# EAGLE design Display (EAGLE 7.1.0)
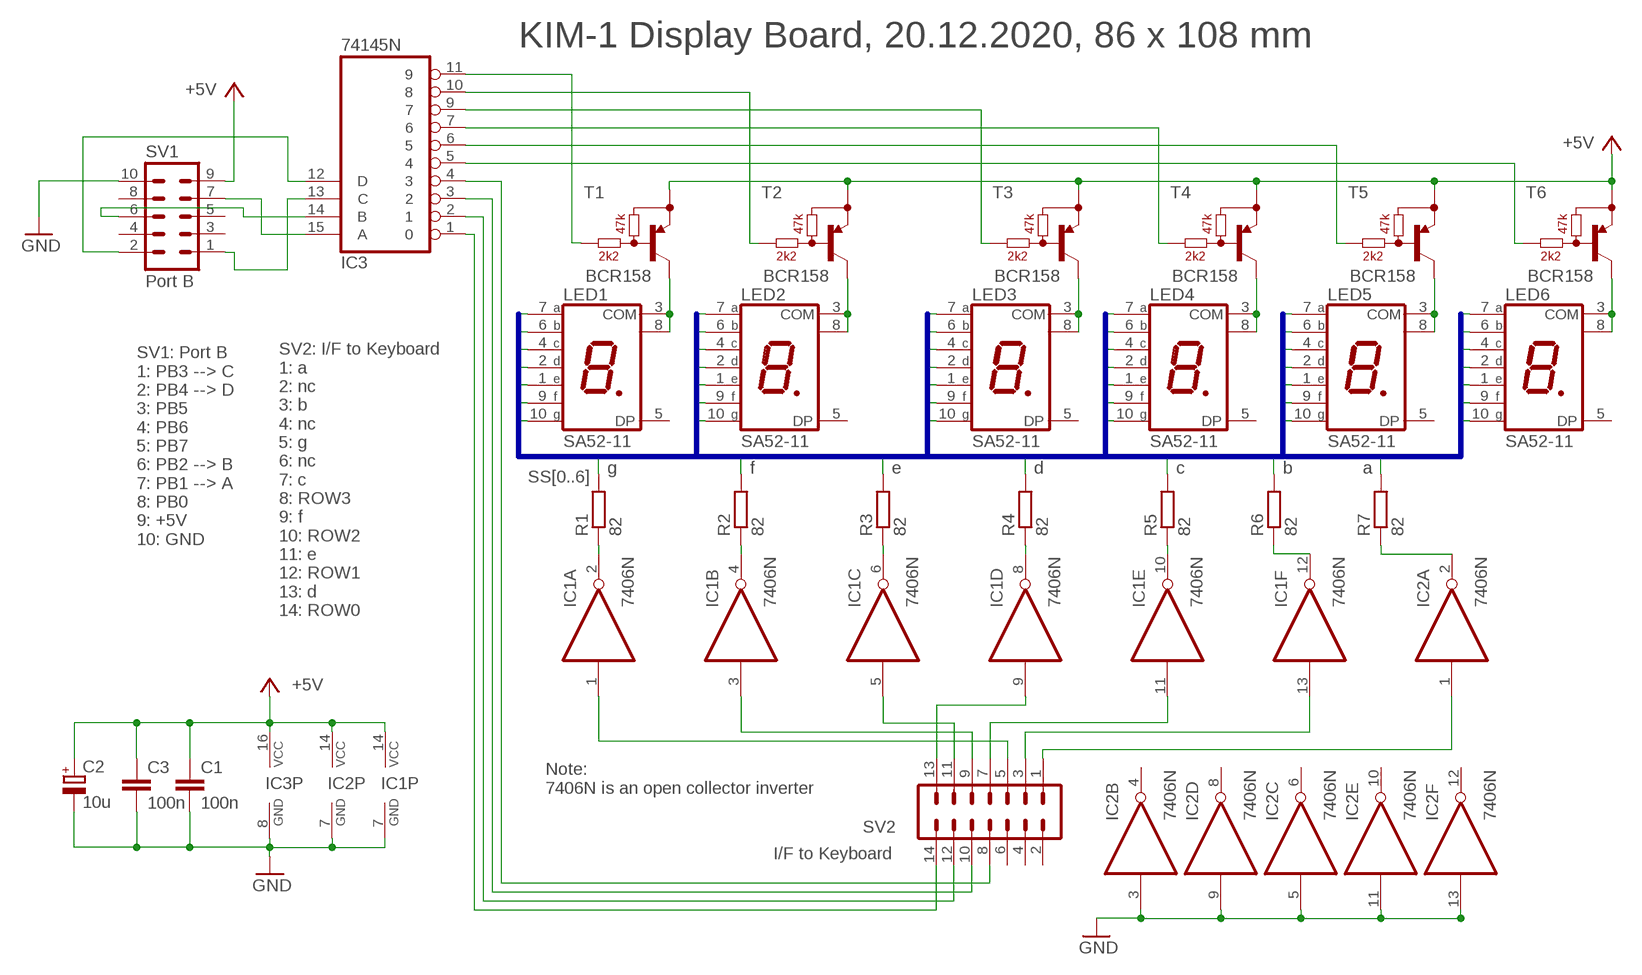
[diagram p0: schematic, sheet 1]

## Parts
C1  100n  C-EUC1206  [C1206]
C2  10u  CPOL-EUE2.5-6  [E2,5-6]
C3  100n  C-EUC1206  [C1206]
IC1  7406N  [DIL14]
IC2  7406N  [DIL14]
IC3  74145N  [DIL16]
LED1  SA52-11  7-SEG_SA52-11  [SA52-11]
LED2  SA52-11  7-SEG_SA52-11  [SA52-11]
LED3  SA52-11  7-SEG_SA52-11  [SA52-11]
LED4  SA52-11  7-SEG_SA52-11  [SA52-11]
LED5  SA52-11  7-SEG_SA52-11  [SA52-11]
LED6  SA52-11  7-SEG_SA52-11  [SA52-11]
R1  82  R-EU_R1206  [R1206]
R2  82  R-EU_R1206  [R1206]
R3  82  R-EU_R1206  [R1206]
R4  82  R-EU_R1206  [R1206]
R5  82  R-EU_R1206  [R1206]
R6  82  R-EU_R1206  [R1206]
R7  82  R-EU_R1206  [R1206]
SV1  Port B  ML10  [ML10]
SV2  I/F to Keyboard  ML14  [ML14]
T1  BCR158  BCR158-W  [SOT23-W_INFINEON]
T2  BCR158  BCR158-W  [SOT23-W_INFINEON]
T3  BCR158  BCR158-W  [SOT23-W_INFINEON]
T4  BCR158  BCR158-W  [SOT23-W_INFINEON]
T5  BCR158  BCR158-W  [SOT23-W_INFINEON]
T6  BCR158  BCR158-W  [SOT23-W_INFINEON]

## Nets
+5V: C1.1 C2.+ C3.1 IC1.14(P:VCC) IC2.14(P:VCC) IC3.16(VCC) SV1.9 T1.2(E) T2.2(E) T3.2(E) T4.2(E) T5.2(E) T6.2(E)
GND: C1.2 C2.- C3.2 IC1.7(P:GND) IC2.3(B:I) IC2.5(C:I) IC2.7(P:GND) IC2.9(D:I) IC2.11(E:I) IC2.13(F:I) IC3.8(GND) SV1.10
N$1: LED6.3(COM) LED6.8(COM) T6.3(C)
N$2: LED5.3(COM) LED5.8(COM) T5.3(C)
N$3: LED3.3(COM) LED3.8(COM) T3.3(C)
N$4: LED2.3(COM) LED2.8(COM) T2.3(C)
N$5: LED1.3(COM) LED1.8(COM) T1.3(C)
N$6: LED4.3(COM) LED4.8(COM) T4.3(C)
N$7: IC1.2(A:O) R1.1
N$8: IC1.4(B:O) R2.1
N$9: IC1.6(C:O) R3.1
N$10: IC1.8(D:O) R4.1
N$11: IC1.10(E:O) R5.1
N$12: IC1.12(F:O) R6.1
N$13: IC2.2(A:O) R7.1
N$14: IC3.11 T1.1(B)
N$15: IC3.10 T2.1(B)
N$16: IC3.9 T3.1(B)
N$17: IC3.7 T4.1(B)
N$18: IC3.6 T5.1(B)
N$19: IC3.5 T6.1(B)
N$20: IC1.1(A:I) SV2.5
N$21: IC1.3(B:I) SV2.9
N$22: IC1.5(C:I) SV2.11
N$23: IC1.9(D:I) SV2.13
N$24: IC1.11(E:I) SV2.7
N$25: IC1.13(F:I) SV2.3
N$26: IC2.1(A:I) SV2.1
N$27: IC3.1 SV2.14
N$28: IC3.2 SV2.12
N$29: IC3.3 SV2.10
N$30: IC3.4 SV2.8
N$31: IC3.15(A) SV1.7
N$36: IC3.14(B) SV1.6
N$37: IC3.13(C) SV1.1
N$38: IC3.12(D) SV1.2
SS0: LED1.7(A) LED2.7(A) LED3.7(A) LED4.7(A) LED5.7(A) LED6.7(A) R7.2
SS1: LED1.6(B) LED2.6(B) LED3.6(B) LED4.6(B) LED5.6(B) LED6.6(B) R6.2
SS2: LED1.4(C) LED2.4(C) LED3.4(C) LED4.4(C) LED5.4(C) LED6.4(C) R5.2
SS3: LED1.2(D) LED2.2(D) LED3.2(D) LED4.2(D) LED5.2(D) LED6.2(D) R4.2
SS4: LED1.1(E) LED2.1(E) LED3.1(E) LED4.1(E) LED5.1(E) LED6.1(E) R3.2
SS5: LED1.9(F) LED2.9(F) LED3.9(F) LED4.9(F) LED5.9(F) LED6.9(F) R2.2
SS6: LED1.10(G) LED2.10(G) LED3.10(G) LED4.10(G) LED5.10(G) LED6.10(G) R1.2
Unconnected: IC2.4(B:O) IC2.6(C:O) IC2.8(D:O) IC2.10(E:O) IC2.12(F:O) LED1.5(DP) LED2.5(DP) LED3.5(DP) LED4.5(DP) LED5.5(DP) LED6.5(DP) SV1.3 SV1.4 SV1.5 SV1.8 SV2.2 SV2.4 SV2.6

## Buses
SS[0..6]

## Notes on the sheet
- KIM-1 Display Board, 20.12.2020, 86 x 108 mm
- g | f | e | d | c | b | a
- SV1: Port B
  1: PB3 --> C
  2: PB4 --> D
  3: PB5
  4: PB6
  5: PB7
  6: PB2 --> B
  7: PB1 --> A
  8: PB0
  9: +5V
  10: GND
- SV2: I/F to Keyboard
  1: a
  2: nc
  3: b
  4: nc
  5: g
  6: nc
  7: c
  8: ROW3
  9: f
  10: ROW2
  11: e
  12: ROW1
  13: d
  14: ROW0
- Note:
  7406N is an open collector inverter

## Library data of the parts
C1 C3 = rcl:C-EU: CAPACITOR, European symbol
C2 = rcl:CPOL-EU: POLARIZED CAPACITOR, European symbol
IC1 IC2 = 74xx-eu:74*06: Hex INVERTER, open collector high-voltage output
IC3 = 74xx-eu:74*145: BCD to decimal DECODER/DRIVER
LED1-LED6 = display-kingbright:7-SEG_: Kingbright 14.2mm (0.56 INCH) SINGLE DIGIT NUMERIC DUISPLAY Source: SA56-11EWA(Ver1189471036.pdf; OC_FARNELL: unknown; OC_NEWARK: unknown
R1-R7 = rcl:R-EU_: RESISTOR, European symbol
SV1 = con-harting-ml:ML10: HARTING; OC_FARNELL: unknown; OC_NEWARK: unknown
SV2 = con-harting-ml:ML14: HARTING; OC_FARNELL: unknown; OC_NEWARK: unknown
T1-T6 = digital-transistors-1:BCR158: PNP Silicon Digital Transistor 50V 0,1A 0,2W

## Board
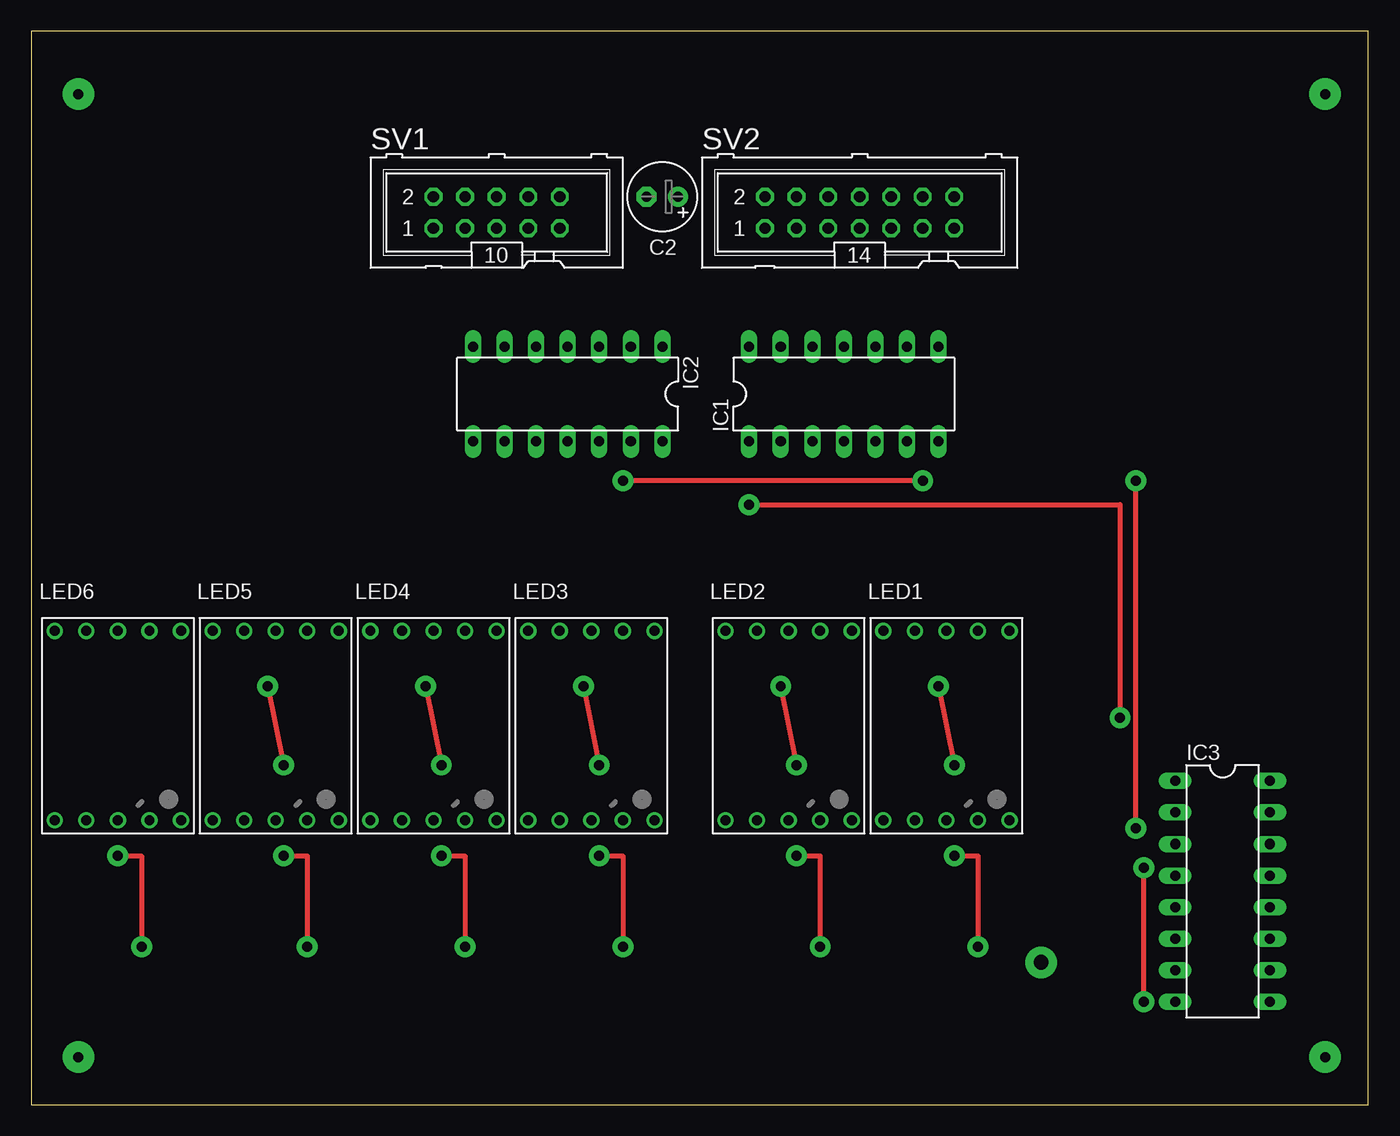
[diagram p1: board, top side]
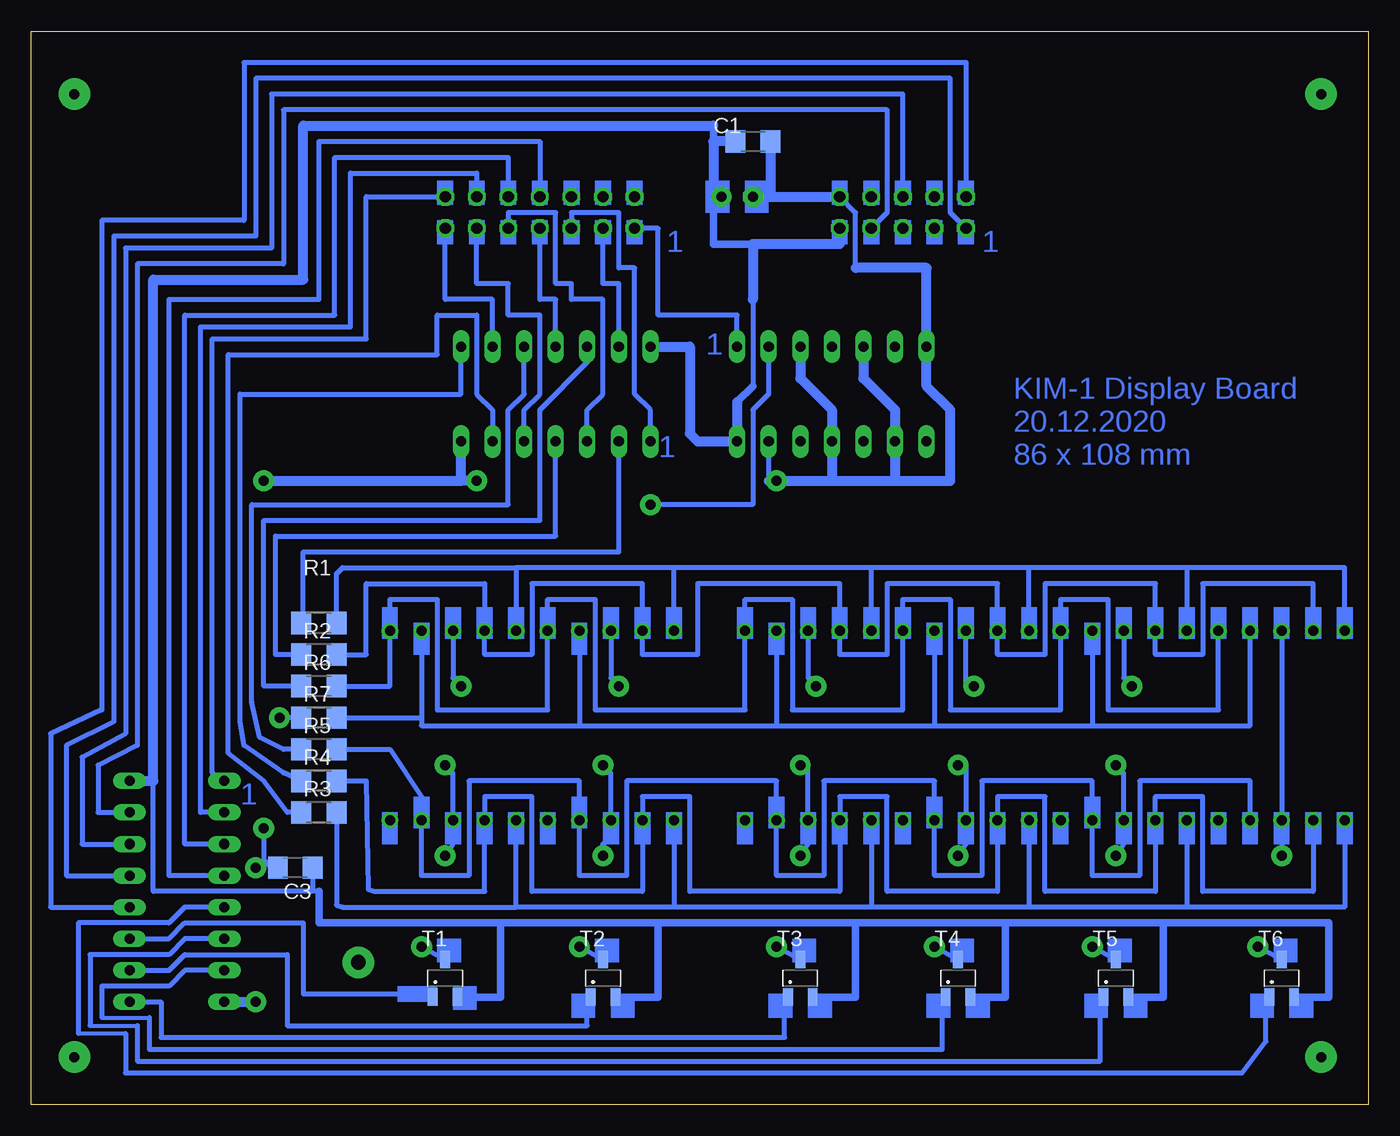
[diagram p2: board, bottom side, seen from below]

Size 107.62 x 86.35 mm. Coordinates in mm from the lower left corner, seen from the top.
Outline: 0,0 107.62,0 107.62,86.35 0,86.35 0,0
Copper layers (1*16): Top 0.035mm / dielectric 1.5mm / Bottom 0.035mm
Design rules "default": minimum track width 10mil, minimum drill 24mil, track to track 8mil, track to pad 8mil, pad to pad 8mil, via to via 8mil, smd to smd 8mil, copper to edge 40mil, drill to drill 8mil, minimum pad ring 10mil, minimum via ring 8mil, stop-mask expansion 4mil, vias tented up to drill 0mil, thermal gap 10mil

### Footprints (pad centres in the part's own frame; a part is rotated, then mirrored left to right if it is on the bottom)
C1206 = smd 1.6 x 1.8: 1 -1.4,0; 2 1.4,0
E2,5-6 = drill 0.813 pad 1.6: + -1.27,0 | drill 0.813 pad 1.6 octagon: - 1.27,0
DIL14 = drill 0.813 long: 1 -7.62,-3.81; 2 -5.08,-3.81; 3 -2.54,-3.81; 4 0,-3.81; 5 2.54,-3.81; 6 5.08,-3.81; 7 7.62,-3.81; 8 7.62,3.81; 9 5.08,3.81; 10 2.54,3.81; 11 0,3.81; 12 -2.54,3.81; 13 -5.08,3.81; 14 -7.62,3.81
DIL16 = drill 0.813 long: 1 -8.89,-3.81; 2 -6.35,-3.81; 3 -3.81,-3.81; 4 -1.27,-3.81; 5 1.27,-3.81; 6 3.81,-3.81; 7 6.35,-3.81; 8 8.89,-3.81; 9 8.89,3.81; 10 6.35,3.81; 11 3.81,3.81; 12 1.27,3.81; 13 -1.27,3.81; 14 -3.81,3.81; 15 -6.35,3.81; 16 -8.89,3.81
SA52-11 = drill 0.8: 1 -5.08,-7.62; 2 -2.54,-7.62; 3 0,-7.62; 4 2.54,-7.62; 5 5.08,-7.62; 6 5.08,7.62; 7 2.54,7.62; 8 0,7.62; 9 -2.54,7.62; 10 -5.08,7.62
R1206 = smd 1.6 x 1.803: 1 -1.422,0; 2 1.422,0
ML10 = drill 0.914 octagon: 1 -5.08,-1.27; 2 -5.08,1.27; 3 -2.54,-1.27; 4 -2.54,1.27; 5 0,-1.27; 6 0,1.27; 7 2.54,-1.27; 8 2.54,1.27; 9 5.08,-1.27; 10 5.08,1.27
ML14 = drill 0.914 octagon: 1 -7.62,-1.27; 2 -7.62,1.27; 3 -5.08,-1.27; 4 -5.08,1.27; 5 -2.54,-1.27; 6 -2.54,1.27; 7 0,-1.27; 8 0,1.27; 9 2.54,-1.27; 10 2.54,1.27; 11 5.08,-1.27; 12 5.08,1.27; 13 7.62,-1.27; 14 7.62,1.27
SOT23-W_INFINEON = smd 0.8 x 1.4: 1 -1,-1.5; 2 1,-1.5; 3 0,1.5

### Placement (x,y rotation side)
C1  49.53,77.47 0 bottom
C2  50.8,73.03 180 top
C3  86.36,19.05 180 bottom
IC1  65.41,57.15 0 top
IC2  43.18,57.15 180 top
IC3  95.89,17.14 270 top
LED1  73.66,30.48 0 top
LED2  60.96,30.48 0 top
LED3  45.09,30.48 0 top
LED4  32.38,30.48 0 top
LED5  19.68,30.48 0 top
LED6  6.99,30.48 0 top
R1  84.45,38.73 0 bottom
R2  84.45,36.2 0 bottom
R3  84.45,23.5 0 bottom
R4  84.45,26.04 0 bottom
R5  84.45,28.57 0 bottom
R6  84.45,33.66 0 bottom
R7  84.45,31.11 0 bottom
SV1  37.47,71.75 0 top
SV2  66.67,71.75 0 top
T1  74.3,10.16 0 bottom
T2  61.59,10.16 0 bottom
T3  45.72,10.16 0 bottom
T4  33.02,10.16 0 bottom
T5  20.32,10.16 0 bottom
T6  6.99,10.16 0 bottom

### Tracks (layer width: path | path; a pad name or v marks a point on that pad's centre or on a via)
+5V
  Bottom 0.406: T6.2 5.99,8.62 | T1.2 73.3,8.62 | T2.2 60.59,8.62 | T5.2 18.68,8.62 | T4.2 31.39,8.62 | T3.2 44.72,8.62 | 51.44,53.34 IC2.14 | 49.53,64.77 49.53,57.78 | 84.45,17.14 85.09,17.14 | 85.09,17.14 97.79,17.14 97.79,26.04 | C3.1 84.96,17.27 85.09,17.14
  Bottom 0.61: 5.99,8.62 3.17,8.62 3.17,14.61 16.51,14.61 | 16.51,14.61 29.21,14.61 | 29.21,14.61 41.27,14.61 | 41.27,14.61 57.15,14.61 | 57.15,14.61 69.85,14.61 | 73.3,8.62 69.85,8.62 69.85,14.61 | 60.59,8.62 57.15,8.62 57.15,14.61 | 18.68,8.62 16.51,8.62 16.51,14.61 | 31.39,8.62 29.21,8.62 29.21,14.61 | 44.72,8.62 41.27,8.62 41.27,14.61 | 69.85,14.61 84.45,14.61 84.45,17.14 | 52.7,78.74 52.7,77.47 | 49.53,69.22 52.7,69.22 52.7,73.03 C2.+ | 49.53,57.78 50.8,56.52 | 50.8,53.98 51.44,53.34
  Bottom 0.813: IC3.16 97.79,26.04 97.79,66.36 85.72,66.36 85.72,78.74 52.7,78.74 | 52.7,73.03 52.7,77.47 C1.1 | 49.53,64.77 49.53,69.22 42.55,69.22 SV1.9 | IC1.14 54.61,60.96 54.61,53.98 53.98,53.34 51.44,53.34 | 50.8,56.52 50.8,53.98
GND  (via drill 0.8 pad 1.68)
  Top 0.406: v71.75,50.16 v47.62,50.16 | v89.53,8.26 v89.53,19.05 | v88.9,22.23 v88.9,50.16
  Bottom 0.406: IC2.13 48.26,50.16 | 41.27,67.31 41.27,71.75 SV1.10 | v88.9,22.23 88.9,19.68 | 88.9,19.68 v89.53,19.05 | C3.2 88.27,19.05 88.9,19.68
  Bottom 0.61: C2.- 48.26,73.03 48.13,73.16
  Bottom 0.813: v88.9,50.16 73.03,50.16 | 73.03,50.16 IC1.7 | IC3.8 v89.53,8.26 | v71.75,50.16 73.03,50.16 | 43.18,50.16 v47.62,50.16 48.26,50.16 | 43.18,50.16 38.1,50.16 | 38.1,50.16 33.66,50.16 33.66,55.88 35.56,57.78 IC2.7 35.56,67.31 41.27,67.31 | 48.26,73.03 SV1.10 | C1.2 48.13,73.16 | 43.18,50.16 IC2.11 43.18,55.88 45.72,58.42 IC2.3 | 38.1,50.16 IC2.9 38.1,55.88 40.64,58.42 IC2.5
N$1  (via drill 0.8 pad 1.68)
  Top 0.406: v6.99,20 8.89,20 v8.89,12.7
  Bottom 0.406: LED6.8 LED6.3 v6.99,20 | T6.3 v8.89,12.7
N$2  (via drill 0.8 pad 1.68)
  Top 0.406: v19.05,33.66 v20.32,27.3 | v20.32,20 22.23,20 v22.23,12.7
  Bottom 0.406: LED5.8 19.68,34.29 19.05,34.29 v19.05,33.66 | v20.32,27.3 20.32,26.67 19.68,26.67 LED5.3 19.68,20.95 v20.32,20 | T5.3 v22.23,12.7
N$3  (via drill 0.8 pad 1.68)
  Top 0.406: v44.45,33.66 v45.72,27.3 | v45.72,20 47.62,20 v47.62,12.7
  Bottom 0.406: LED3.8 45.09,34.29 44.45,34.29 v44.45,33.66 | v45.72,27.3 45.09,27.3 LED3.3 45.09,20.95 v45.72,20 | T3.3 v47.62,12.7
N$4  (via drill 0.8 pad 1.68)
  Top 0.406: v60.33,33.66 v61.59,27.3 | v61.59,20 63.5,20 v63.5,12.7
  Bottom 0.406: v61.59,27.3 61.59,26.67 60.96,26.67 LED2.3 60.96,21.59 61.59,20.95 v61.59,20 | LED2.8 60.96,34.29 60.33,34.29 v60.33,33.66 | T2.3 v63.5,12.7
N$5  (via drill 0.8 pad 1.68)
  Top 0.406: v73.03,33.66 v74.3,27.3 | v74.3,20 76.2,20 v76.2,12.7
  Bottom 0.406: LED1.8 73.66,34.29 73.03,34.29 v73.03,33.66 | v74.3,27.3 74.3,26.67 73.66,26.67 LED1.3 73.66,20.95 v74.3,20 | T1.3 v76.2,12.7
N$6  (via drill 0.8 pad 1.68)
  Top 0.406: v31.75,33.66 v33.02,27.3 | v33.02,20 34.92,20 v34.92,12.7
  Bottom 0.406: v31.75,33.66 32.38,33.66 LED4.8 | v33.02,27.3 32.38,27.3 LED4.3 32.38,20.95 v33.02,20 | T4.3 v34.92,12.7
N$7
  Bottom 0.406: R1.1 85.72,38.73 85.72,44.45 60.33,44.45 IC1.2
N$8
  Bottom 0.406: R2.1 87.95,36.2 87.95,45.72 65.41,45.72 IC1.4
N$9
  Bottom 0.406: R3.1 87,23.5 88.9,26.04 91.76,28.26 91.76,60.33 74.93,60.33 74.93,63.5 71.75,63.5 71.75,57.15 70.48,55.88 IC1.6
N$10
  Bottom 0.406: R4.1 87.31,26.67 90.49,28.89 90.81,30.8 90.81,57.15 73.03,57.15 IC1.8
N$11
  Bottom 0.406: R5.1 87.31,28.57 89.22,29.53 89.85,32.38 89.85,48.26 69.22,48.26 69.22,55.88 67.94,57.15 IC1.10
N$12
  Bottom 0.406: R6.1 88.9,33.66 88.9,46.99 66.67,46.99 66.67,55.88 62.87,59.69 IC1.12
N$13  (via drill 0.8 pad 1.68)
  Top 0.406: v57.78,48.26 87.63,48.26 v87.63,31.11
  Bottom 0.406: R7.1 v87.63,31.11 | IC2.2 48.26,57.15 49.53,55.88 49.53,48.26 v57.78,48.26
N$14
  Bottom 0.406: IC3.11 96.52,13.34 95.25,14.61 85.72,14.61 85.72,8.89 75.53,8.89 T1.1
N$15
  Bottom 0.406: IC3.10 96.52,10.79 95.25,12.06 87,12.06 87,6.35 62.87,6.35 62.87,8.39 T2.1
N$16
  Bottom 0.406: IC3.9 97.16,8.26 97.16,5.4 46.99,5.4 46.99,8.39 T3.1
N$17
  Bottom 0.305: 101.92,6.99 98.11,6.99
  Bottom 0.406: IC3.7 95.25,10.79 96.52,9.53 101.92,9.53 101.92,6.99 | 98.11,6.99 98.11,4.45 34.29,4.45 34.29,8.39 T4.1
N$18
  Bottom 0.305: 102.87,6.35 99.06,6.35
  Bottom 0.406: IC3.6 95.25,13.34 96.52,12.06 102.87,12.06 102.87,6.35 | 99.06,6.35 99.06,3.49 21.59,3.49 21.59,8.39 T5.1
N$19
  Bottom 0.305: 103.82,5.71 100.01,5.71
  Bottom 0.406: IC3.5 95.25,15.88 96.52,14.61 103.82,14.61 103.82,5.71 | 100.01,5.71 100.01,2.54 10.16,2.54 8.26,5.08 8.26,8.39 T6.1
N$20
  Bottom 0.406: IC1.1 57.78,55.88 59.05,57.15 59.05,67.31 60.33,67.31 60.33,71.75 64.14,71.75 SV2.5
N$21
  Bottom 0.406: IC1.3 62.87,55.88 61.59,57.15 61.59,64.77 64.14,64.77 64.14,66.04 65.41,66.04 65.41,71.75 69.22,71.75 SV2.9
N$22
  Bottom 0.406: IC1.5 67.94,55.88 66.67,57.15 66.67,63.5 69.22,63.5 69.22,66.04 71.75,66.04 SV2.11
N$23
  Bottom 0.406: IC1.9 70.48,64.77 74.3,64.77 SV2.13
N$24
  Bottom 0.406: IC1.11 65.41,64.77 66.67,64.77 SV2.7
N$25
  Bottom 0.406: IC1.13 60.33,66.04 61.59,66.04 SV2.3
N$26
  Bottom 0.406: IC2.1 50.8,63.5 57.15,63.5 57.15,70.48 SV2.1
N$27
  Bottom 0.406: IC3.1 93.03,26.67 93.03,61.59 80.64,61.59 80.64,73.03 SV2.14
N$28
  Bottom 0.406: IC3.2 93.98,23.5 93.98,62.55 81.92,62.55 81.92,74.93 71.75,74.93 SV2.12
N$29
  Bottom 0.406: IC3.3 95.25,20.95 95.25,63.5 83.19,63.5 83.19,76.2 69.22,76.2 SV2.10
N$30
  Bottom 0.406: IC3.4 96.52,18.41 96.52,64.77 84.45,64.77 84.45,77.47 66.67,77.47 SV2.8
N$31
  Bottom 0.406: IC3.15 102.23,23.5 102.23,27.3 99.06,28.89 99.06,67.63 87.31,67.63 87.31,80.01 38.73,80.01 38.73,71.75 SV1.7
N$32  (via drill 0.8 pad 2.54)
  other vias: 3.81,81.28
N$33  (via drill 0.8 pad 2.54)
  other vias: 104.14,81.28
N$34  (via drill 0.8 pad 2.54)
  other vias: 104.14,3.81
N$35  (via drill 0.8 pad 2.54)
  other vias: 3.81,3.81
N$36
  Bottom 0.406: IC3.14 103.5,20.95 103.5,27.94 100.01,29.84 100.01,68.9 88.27,68.9 88.27,81.28 37.47,81.28 SV1.6
N$37
  Bottom 0.406: IC3.13 104.78,18.41 104.78,28.89 100.97,30.8 100.97,69.85 89.53,69.85 89.53,82.55 33.66,82.55 33.66,71.75 SV1.1
N$38
  Bottom 0.406: IC3.12 106.05,15.88 106.05,29.84 101.92,31.75 101.92,71.12 90.49,71.12 90.49,83.82 32.38,83.82 SV1.2
N$39  (via drill 1.2 pad 2.54)
  other vias: 81.28,11.43
SS0
  Bottom 0.406: LED1.7 76.2,31.11 | 76.2,31.11 76.2,30.48 63.5,30.48 | 63.5,30.48 47.62,30.48 | 47.62,30.48 34.92,30.48 | 34.92,30.48 22.23,30.48 | 22.23,30.48 9.53,30.48 LED6.7 | LED5.7 22.23,30.48 | LED4.7 34.92,30.48 | LED3.7 47.62,30.48 | LED2.7 63.5,30.48 | R7.2 76.2,31.11
SS1
  Bottom 0.406: LED6.6 12.06,31.75 20.95,31.75 20.95,40.64 24.77,40.64 LED5.6 24.77,31.75 33.66,31.75 33.66,40.64 37.47,40.64 LED4.6 37.47,31.75 46.35,31.75 46.35,40.64 50.16,40.64 LED3.6 50.16,31.75 62.23,31.75 62.23,40.64 66.04,40.64 LED2.6 66.04,31.75 74.93,31.75 74.93,40.64 78.74,40.64 LED1.6 78.74,33.66 R6.2
SS2
  Bottom 0.406: LED6.4 9.53,26.04 18.41,26.04 18.41,18.41 22.23,18.41 LED5.4 22.23,26.04 31.11,26.04 31.11,18.41 34.92,18.41 LED4.4 34.92,26.04 43.81,26.04 43.81,18.41 47.62,18.41 LED3.4 47.62,26.04 59.69,26.04 59.69,18.41 63.5,18.41 LED2.4 63.5,26.04 72.39,26.04 72.39,18.41 76.2,18.41 LED1.4 76.2,24.77 78.74,28.57 R5.2
SS3
  Bottom 0.406: LED6.2 4.45,17.14 13.34,17.14 13.34,24.77 17.14,24.77 LED5.2 17.14,17.14 26.04,17.14 26.04,24.77 29.84,24.77 LED4.2 29.84,17.14 38.73,17.14 38.73,24.77 42.55,24.77 LED3.2 42.55,17.14 54.61,17.14 54.61,24.77 58.42,24.77 LED2.2 58.42,17.14 67.31,17.14 67.31,24.77 71.12,24.77 LED1.2 71.12,17.14 80.01,17.14 80.49,17.3 80.64,26.04 R4.2
SS4
  Bottom 0.406: LED6.1 1.91,15.88 14.61,15.88 | 14.61,15.88 27.3,15.88 | 27.3,15.88 40.01,15.88 | 40.01,15.88 55.88,15.88 | 55.88,15.88 68.58,15.88 | 68.58,15.88 LED1.1 | LED5.1 14.61,15.88 | LED4.1 27.3,15.88 | LED3.1 40.01,15.88 | LED2.1 55.88,15.88 | R3.2 83.03,16.04 82.55,15.88 68.58,15.88
SS5
  Bottom 0.406: LED6.9 4.45,41.91 13.34,41.91 13.34,36.2 17.14,36.2 LED5.9 17.14,41.91 26.04,41.91 26.04,36.2 29.84,36.2 LED4.9 29.84,41.91 38.73,41.91 38.73,36.2 42.55,36.2 LED3.9 42.55,41.91 53.98,41.91 53.98,36.2 58.42,36.2 LED2.9 58.42,41.91 67.31,41.91 67.31,36.2 71.12,36.2 LED1.9 71.12,41.91 80.64,41.91 80.64,36.2 R2.2
SS6
  Bottom 0.406: LED6.10 1.91,43.18 14.61,43.18 | 14.61,43.18 LED5.10 | LED4.10 27.3,43.18 | 27.3,43.18 40.01,43.18 | 40.01,43.18 55.88,43.18 | 55.88,43.18 68.58,43.18 | 68.58,43.18 LED1.10 | LED2.10 55.88,43.18 | LED3.10 40.01,43.18 | 14.61,43.18 27.3,43.18 | R1.2 83.03,42.7 82.55,43.18 68.58,43.18
(copper drawn outside any net)
  shapes: Bottom area x104

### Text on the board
Bottom: 1 | 1 | 1 | 1 | KIM-1 Display Board / 20.12.2020 / 86 x 108 mm | 1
